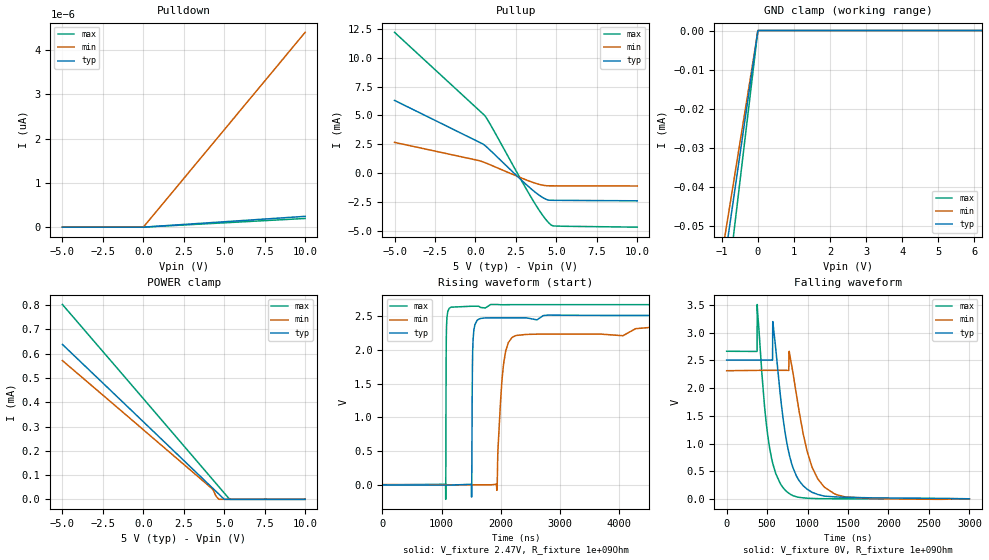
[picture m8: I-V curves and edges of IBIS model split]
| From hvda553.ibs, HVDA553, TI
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|   split Model
[Model]   split
Model_type   3-state
Polarity   Inverting
Vmeas = 1.25
Vref = 2.47
Cref = 100pF
Rref = 1e9
|   typ   min   max
|   (nom PVT)   (fast PVT)   (slow PVT)
C_comp   2.229e-11   1.633e-11   4.612e-11
| Where nom  PVT is Nominal Process, 5V, 27C
|   Fast PVT is Strong Process,  5.33V, -40C
|   Slow PVT is Weak Process,   4.68V, 150C
[Voltage Range]   5   4.68   5.33
|Junction Temperature
[Temperature Range]   27   150   -40
[Pullup Reference]   5   4.68   5.33
[Pulldown Reference]   0   0   0
[Power Clamp Reference]   5   4.68   5.33
[GND Clamp Reference]   0   0   0
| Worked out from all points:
|   slope of the pullup table from 0 to 0.75 V, typ, clamps not added: 1.15 kohm
|   rising waveform, V_fixture 2.47V, R_fixture 1e+09Ohm: 20-80 % time 14.2ns typ, 110ns min, 6.71ns max; typ from 0.003 V to 2.51 V
|   falling waveform, V_fixture 0V, R_fixture 1e+09Ohm: 20-80 % time 182ns typ, 226ns min, 148ns max; typ from 2.51 V to 0.004 V
[Pulldown]
|   Voltage   I(typ)   I(min)   I(max)
-5V       0A         0A         0A
0V        0A         0A         0A
9.995V    244fA      4.4pA      196.2fA
[GND Clamp]
|   Voltage   I(typ)   I(min)   I(max)
-5V       -319.4uA   -287.2uA   -388.7uA
-1.674V   -107uA     -96.24uA   -130.2uA
-500mV    -32.08uA   -28.99uA   -39.02uA
-460uV    -200nA     -205.5nA   -238.2nA
2.92mV    -120.8nA   0A         -162.7nA
10mV      0A         0A         0A
9.995V    0A         0A         0A
[Pullup]
|   Voltage   I(typ)   I(min)   I(max)
-5V       6.303mA    2.66mA     12.21mA
100.8mV   2.768mA    1.113mA    5.599mA
596.5mV   2.376mA    893.7uA    4.939mA
930mV     1.948mA    699.6uA    4.182mA
2.942V    -751uA     -492.2uA   -902.2uA
3.565V    -1.524mA   -825.3uA   -2.406mA
4.258V    -2.209mA   -1.082mA   -3.875mA
4.653V    -2.365mA   -1.112mA   -4.486mA
4.919V    -2.37mA    -1.113mA   -4.601mA
9.995V    -2.412mA   -1.127mA   -4.699mA
[POWER Clamp]
|   Voltage   I(typ)   I(min)   I(max)
-5V       638.1uA    571.5uA    802.6uA
4.182V    52.27uA    47.47uA    89.35uA
4.318V    43.6uA     37.09uA    78.78uA
4.5V      31.93uA    12.83uA    64.58uA
4.678V    20.57uA    84.11nA    50.73uA
5.005V    0A         0A         25.3uA
5.33V     0A         0A         35.27nA
9.995V    0A         0A         0A
[Ramp]
R_load = 1e+09
|   typ   min   max
dV/dt_r   1.5023/1.38725e-08   1.38873/1.08316e-07   1.59769/6.641e-09
dV/dt_f   1.50176/1.80512e-07   1.3875/2.21993e-07   1.59773/1.47897e-07
[Rising Waveform]
V_fixture = 2.47V
V_fixture_min = 2V
V_fixture_max = 2.66V
R_fixture = 1e+09Ohm
|   Time   V(typ)   V(min)   V(max)
0s        3.158mV    7.618mV    3.263mV
1.07us    527.2uV    4.78mV     -210.2mV
1.084us   525.5uV    4.766mV    2.338V
1.162us   516.3uV    4.687mV    2.629V
1.508us   -177.1mV   4.366mV    2.642V
1.533us   2.148V     4.344mV    2.642V
1.627us   2.451V     4.262mV    2.642V
1.936us   2.471V     -77.34mV   2.668V
2.191us   2.471V     2.181V     2.666V
6us       2.507V     2.322V     2.666V
[Falling Waveform]
V_fixture = 0V
V_fixture_min = 0V
V_fixture_max = 0V
R_fixture = 1e+09Ohm
|   Time   V(typ)   V(min)   V(max)
0s        2.507V     2.315V     2.666V
376.5ns   2.507V     2.321V     2.663V
378.4ns   2.507V     2.321V     3.51V
468.7ns   2.507V     2.322V     1.668V
567.4ns   2.504V     2.322V     658.2mV
571ns     3.201V     2.322V     637mV
799ns     661.4mV    2.451V     75.8mV
998.1ns   174mV      843.7mV    14.44mV
1.21us    51.68mV    212.1mV    4.981mV
3us       3.879mV    2.257mV    3.063mV
